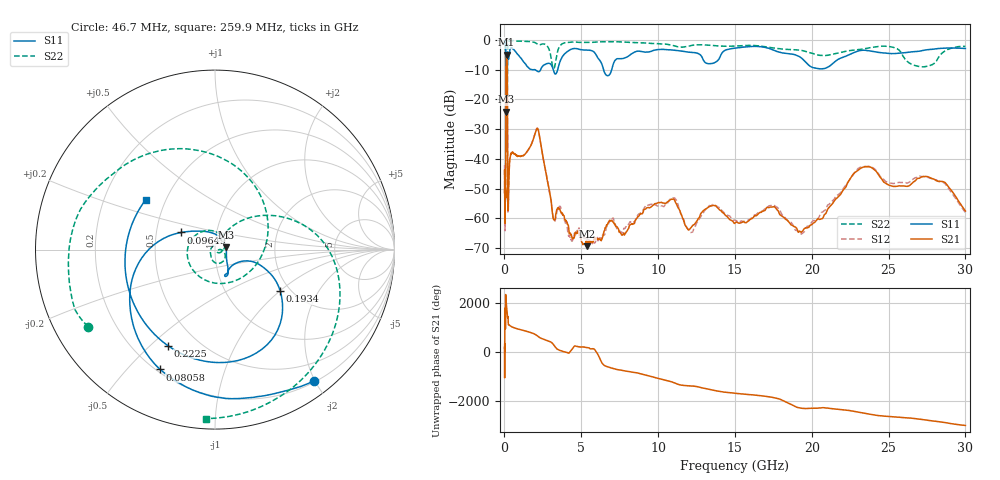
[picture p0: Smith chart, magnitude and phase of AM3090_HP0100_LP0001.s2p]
! Date/Time: Thu, Feb 28, 2019 1:57 PM
! Network Analyzer: Agilent Technologies E8364B Rev: A.07.50.67
! Sweep from 0.010 to 30.000 GHz, 1601 Points, Sweep Type: LOG
! Power Supply: 5.023 V, 0.002 A
# Hz S DB R 50
!freq MagS11 AngS11 MagS21 AngS21 MagS12 AngS12 MagS22 AngS22
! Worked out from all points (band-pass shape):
!   1601 points, 10 MHz to 30 GHz, reference 50 ohm
!   highest |S21| = -4.88 dB at 138.3 MHz (marker M1); lowest = -69.4 dB at 5.392 GHz (marker M2)
!   |S21| within 3 dB of the highest: 104.3 MHz to 178.2 MHz (73.9 MHz wide, 52.3 % of centre)
!   lowest |S11| = -24.1 dB at 103.5 MHz (marker M3), VSWR 1.13, Z = 56.5 + j1.38 ohm
!   |S11| at or under -10 dB: 1.994 GHz to 2.352 GHz (357.3 MHz wide, 16.4 % of centre); 3.18 GHz to 3.465 GHz (285 MHz wide, 8.58 % of centre); 6.454 GHz to 6.979 GHz (525.2 MHz wide, 7.82 % of centre)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
!   |S22| runs from -37.5 to -0.1 dB; largest |S21 - S12| = 0.013
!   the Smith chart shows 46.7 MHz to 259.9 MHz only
!   S11 on the Smith chart (normalised r, x): 46.7 MHz: 0.22, -1.98; 80.58 MHz: 0.21, -0.62; 96.49 MHz: 0.67, +0.13; 193.4 MHz: 1.77, -1.01; 222.5 MHz: 0.34, -0.57; 259.9 MHz: 0.39, +0.28
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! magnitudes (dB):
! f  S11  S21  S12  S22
! 10 MHz  -0.2  -45.1  -42.1  -0.5
! 38.04 MHz  -0.5  -59.3  -62.2  -1.3
! 46.7 MHz  -0.8  -50.5  -51.6  -1.6
! 80.58 MHz  -2.7  -46.3  -46.0  -5.6
! 96.49 MHz  -13.5  -14.1  -14.1  -15.2
! 103.5 MHz  -24.1  -8.2  -8.2  -17.4
! 138.3 MHz  -16.6  -4.9  -4.8  -31.8
! 144.7 MHz  -16.6  -4.9  -4.9  -24.1
! 171.5 MHz  -16.0  -6.6  -6.5  -33.0
! 193.4 MHz  -7.3  -19.1  -19.0  -9.6
! 222.5 MHz  -4.5  -57.5  -57.5  -1.4
! 259.9 MHz  -6.5  -55.2  -53.0  -0.5
! 335.4 MHz  -3.8  -40.9  -40.9  -0.2
! 550.5 MHz  -3.0  -37.9  -38.1  -0.2
! 2.084 GHz  -10.3  -30.1  -30.0  -1.2
! 3.22 GHz  -10.7  -60.4  -60.3  -9.6
! 5.392 GHz  -3.4  -69.4  -66.6  -0.8
! 7.926 GHz  -5.8  -64.6  -62.8  -0.7
! 10.65 GHz  -3.3  -54.4  -54.5  -1.5
! 19.51 GHz  -6.9  -63.5  -64.6  -3.7
! 23.48 GHz  -3.4  -42.6  -42.6  -2.9
! 30 GHz  -2.8  -57.5  -58.1  -2.1
